{attribute 'no_assign'}
{attribute 'call_after_init'}
FUNCTION_BLOCK FB_DS_IED_MUnn_LLN0_PhsMeas1 EXTENDS FB_AcsiCommonDataSetClass
VAR
END_VAR

METHOD OnInit : BOOL
VAR
END_VAR
IF NOT DeleteAllMembers() THEN RETURN; END_IF
IF NOT AddMember(ipData:=fbIED.IEDMUnn.InnATCTR1.AmpSv, eFc:=E_AcsiFc.MX) THEN RETURN; END_IF
IF NOT AddMember(ipData:=fbIED.IEDMUnn.InnBTCTR2.AmpSv, eFc:=E_AcsiFc.MX) THEN RETURN; END_IF
IF NOT AddMember(ipData:=fbIED.IEDMUnn.InnCTCTR3.AmpSv, eFc:=E_AcsiFc.MX) THEN RETURN; END_IF
IF NOT AddMember(ipData:=fbIED.IEDMUnn.InnNTCTR4.AmpSv, eFc:=E_AcsiFc.MX) THEN RETURN; END_IF
IF NOT AddMember(ipData:=fbIED.IEDMUnn.UnnATVTR1.VolSv, eFc:=E_AcsiFc.MX) THEN RETURN; END_IF
IF NOT AddMember(ipData:=fbIED.IEDMUnn.UnnBTVTR2.VolSv, eFc:=E_AcsiFc.MX) THEN RETURN; END_IF
IF NOT AddMember(ipData:=fbIED.IEDMUnn.UnnCTVTR3.VolSv, eFc:=E_AcsiFc.MX) THEN RETURN; END_IF
IF NOT AddMember(ipData:=fbIED.IEDMUnn.UnnNTVTR4.VolSv, eFc:=E_AcsiFc.MX) THEN RETURN; END_IF
OnInit:= TRUE;
END_METHOD

END_FUNCTION_BLOCK
